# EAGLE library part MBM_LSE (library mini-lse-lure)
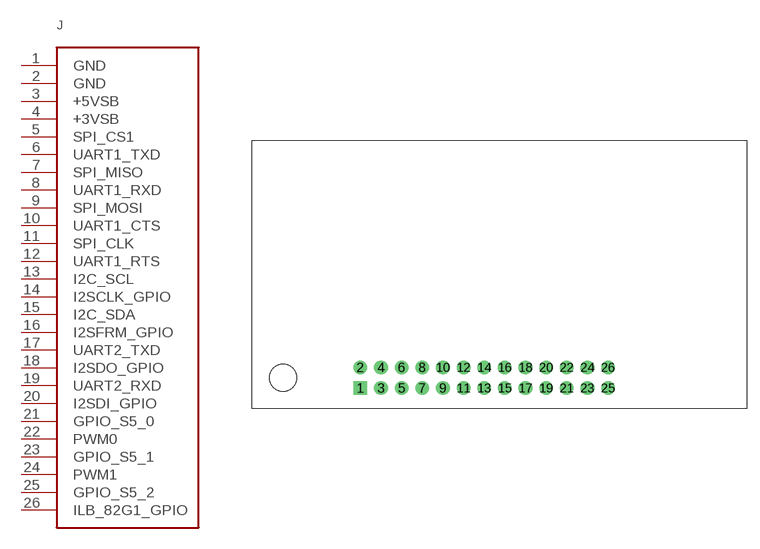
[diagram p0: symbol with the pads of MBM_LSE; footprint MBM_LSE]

Designator prefix J

## MBM_LSE  [MBM_LSE]
1  GND
2  GND
3  +5VSB
4  +3VSB
5  SPI_CS1
6  UART1_TXD
7  SPI_MISO
8  UART1_RXD
9  SPI_MOSI
10  UART1_CTS
11  SPI_CLK
12  UART1_RTS
13  I2C_SCL
14  I2SCLK_GPIO
15  I2C_SDA
16  I2SFRM_GPIO
17  UART2_TXD
18  I2SDO_GPIO
19  UART2_RXD
20  I2SDI_GPIO
21  GPIO_S5_0
22  PWM0
23  GPIO_S5_1
24  PWM1
25  GPIO_S5_2
26  ILB_82G1_GPIO

## Footprint MBM_LSE (pad centres in mm)
drill 1.1 pad 1.676 square: 1 -15.24,0
drill 1.1 pad 1.676: 2 -15.24,2.54; 3 -12.7,0; 4 -12.7,2.54; 5 -10.16,0; 6 -10.16,2.54; 7 -7.62,0; 8 -7.62,2.54; 9 -5.08,0; 10 -5.08,2.54; 11 -2.54,0; 12 -2.54,2.54; 13 0,0; 14 0,2.54; 15 2.54,0; 16 2.54,2.54; 17 5.08,0; 18 5.08,2.54; 19 7.62,0; 20 7.62,2.54; 21 10.16,0; 22 10.16,2.54; 23 12.7,0; 24 12.7,2.54; 25 15.24,0; 26 15.24,2.54
hole 3.302 at -24.765,1.27

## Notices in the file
Licensing: Creative Commons Attribution Share-Alike 3.0 License http://creativecommons.org/licenses/by-sa/3.0
